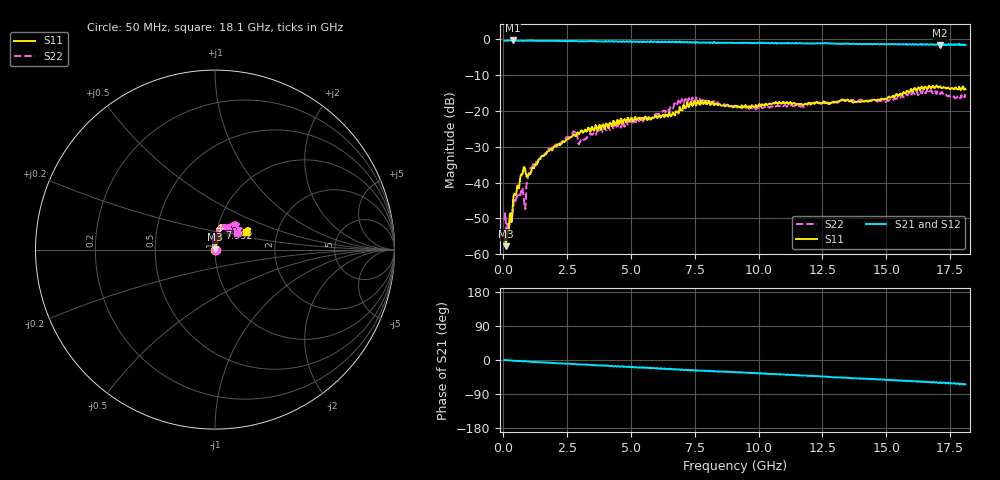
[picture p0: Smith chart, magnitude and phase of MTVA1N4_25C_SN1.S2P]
! Network Analyzer HP8720D.06.14 Serial No. US36140669
! 12 Jan 2005  08:39:05
! Frequency  S11  S21  S12  S22
# HZ  S  DB R 50
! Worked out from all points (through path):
!   801 points, 50 MHz to 18.1 GHz, reference 50 ohm
!   highest |S21| = -0.37 dB at 365.9 MHz (marker M1); lowest = -1.7 dB at 17.11 GHz (marker M2)
!   group delay of S21, straight-line fit = 9.5 ps
!   lowest |S11| = -57.7 dB at 95.12 MHz (marker M3), VSWR 1.00, Z = 50.1 + j0.0804 ohm
!   |S11| at or under -10 dB: start of sweep to end of sweep
!   |S22| runs from -54.2 to -14.2 dB; largest |S21 - S12| = 0.034
!   S11 on the Smith chart (normalised r, x): 50 MHz: 1.00, -0.00; 7.992 GHz: 1.02, +0.26; 18.1 GHz: 1.38, +0.29
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5e7  -56.01 -43.9  -0.41 -0.3  -0.43 -0.6  -50.32 -4.0
9.5125e7  -57.72 38.1  -0.44 -0.6  -0.43 -0.9  -50.60 -5.2
2.079375e8  -54.21 93.2  -0.41 -0.7  -0.40 -1.0  -51.83 36.7
3.65875e8  -47.13 91.8  -0.37 -1.9  -0.36 -2.0  -48.80 62.8
5.238125e8  -42.23 89.8  -0.43 -2.7  -0.41 -2.9  -44.02 72.3
7.494375e8  -37.72 81.8  -0.45 -3.2  -0.45 -3.5  -41.42 69.0
8.6225e8  -36.72 60.5  -0.45 -3.5  -0.44 -4.0  -47.39 124.0
9.97625e8  -37.49 70.3  -0.44 -4.1  -0.41 -4.4  -37.82 111.8
1.110438e9  -36.24 84.0  -0.44 -4.7  -0.39 -4.9  -35.77 106.0
1.448875e9  -33.44 83.2  -0.48 -5.9  -0.46 -6.2  -32.69 103.2
2.802625e9  -26.95 71.3  -0.55 -11.1  -0.53 -11.6  -26.10 99.3
3.073375e9  -25.44 74.8  -0.57 -12.0  -0.53 -12.1  -28.14 97.3
4.043562e9  -23.59 69.0  -0.64 -15.1  -0.56 -15.1  -25.35 95.3
6.074188e9  -21.71 74.1  -0.70 -22.9  -0.70 -22.8  -20.96 83.7
7.066938e9  -18.32 74.7  -0.81 -26.7  -0.76 -26.1  -17.92 70.3
7.992e9  -18.01 77.3  -0.93 -28.6  -0.96 -29.2  -17.27 50.9
9.075e9  -18.62 81.2  -1.06 -32.0  -0.98 -32.5  -18.86 45.1
1.209838e10  -17.94 65.6  -1.18 -42.0  -1.16 -42.4  -17.88 58.4
1.509919e10  -16.01 35.2  -1.37 -52.9  -1.28 -52.6  -17.16 59.6
1.61145e10  -13.58 28.8  -1.61 -56.1  -1.34 -56.3  -15.33 52.4
1.710725e10  -13.26 30.4  -1.72 -59.3  -1.61 -59.5  -15.31 39.6
1.81e10  -13.95 30.1  -1.66 -64.3  -1.65 -65.4  -16.30 38.5
